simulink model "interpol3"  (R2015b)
settings: Solver=VariableStepAuto  StartTime=0.0  StopTime=10.0  RelTol=1e-3
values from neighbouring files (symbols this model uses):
  a = 1/(Tsig/2.5)    (= 7.8125)    [fourier_transf_puls_3.m]    (also in fourier_transf_puls_4.m; schar_1.m = 5)
  b = 10    [schar_1.m]
  hint1 = fir1(nord, 1/L1)    [interpol_3.m]
  hint2 = fir1(nord, 1/L2)    [interpol_3.m]
  L1 = 20    [interpol_3.m]
  L2 = 8    [interpol_3.m]
  nord = 6    [dezimier_1.m]    (also in dezimier_11.m; dezimier_2.m = 256; dezimier_3.m = 256; farrow_2.m = 128)
  Ts = 1/fs    (= 5e-05)    [basisband_1.m]    (also in basisband_2.m = 5e-06; dezimier_1.m = 0.0005; dezimier_11.m = 0.0005; dezimier_2.m = 0.0005)
libraries: dspsigops x2

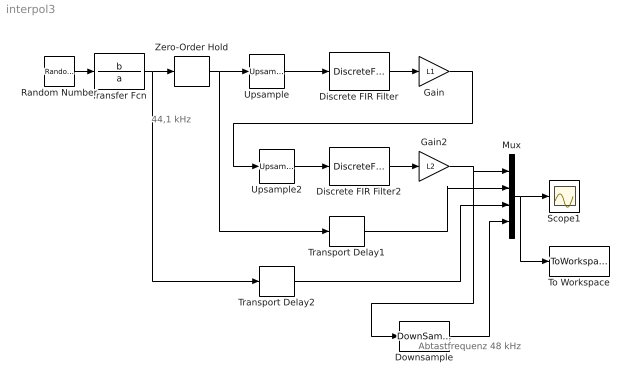
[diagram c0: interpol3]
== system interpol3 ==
  note: Abtastfrequenz 48 kHz
  note: 44,1 kHz
  Discrete FIR Filter : DiscreteFir  Coefficients=hint1
  Discrete FIR Filter2 : DiscreteFir  Coefficients=hint2
  Downsample : DownSample  N=147  RateOptions=Allow multirate processing
  Gain : Gain  Gain=L1
  Gain2 : Gain  Gain=L2
  Mux : Mux
  Random Number : RandomNumber  Seed=03678  SampleTime=0
  Scope1 : Scope
  To Workspace : ToWorkspace  VariableName=y  SaveFormat=Timeseries  SampleTime=-1
  Transfer Fcn : TransferFcn  Numerator=b  Denominator=a
  Transport Delay1 : TransportDelay  DelayTime=(nord/2)*(Ts/L1)*(1+1/L2)  BufferSize=1024*4
  Transport Delay2 : TransportDelay  DelayTime=(nord/2)*(Ts/L1)*(1+1/L2)  BufferSize=1024*4
  Upsample : dspsigops/Upsample  N=L1  phase=0  RateOptions=Allow multirate processing  ic=0  mode=Unused parameter value
  Upsample2 : dspsigops/Upsample  N=L2  phase=0  RateOptions=Allow multirate processing  ic=0  mode=Unused parameter value
  Zero-Order Hold : ZeroOrderHold  SampleTime=Ts
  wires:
  Random Number/1 -> Transfer Fcn/1
  Upsample/1 -> Discrete FIR Filter/1
  Discrete FIR Filter/1 -> Gain/1
  Transfer Fcn/1 -> Transport Delay2/1, Zero-Order Hold/1
  Mux/1 -> Scope1/1, To Workspace/1
  Zero-Order Hold/1 -> Transport Delay1/1, Upsample/1
  Upsample2/1 -> Discrete FIR Filter2/1
  Discrete FIR Filter2/1 -> Gain2/1
  Gain/1 -> Upsample2/1
  Gain2/1 -> Mux/1, Downsample/1
  Transport Delay2/1 -> Mux/3
  Transport Delay1/1 -> Mux/2
  Downsample/1 -> Mux/4
